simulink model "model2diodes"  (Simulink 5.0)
settings: Solver=ode23t  StartTime=0.0  StopTime=24  FixedStep=0.0001  RelTol=1e-3

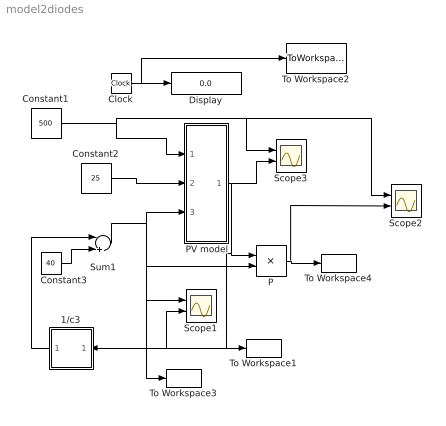
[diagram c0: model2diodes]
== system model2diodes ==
  1/c3 : Subsystem  Orientation=left
  Clock : Clock
  Constant1 : Constant  Value=500
  Constant2 : Constant  Value=25
  Constant3 : Constant  Value=40
  Display : Display
  P : Product
  PV model : Subsystem  mask{p1=0.00345, p2=0.0058e-3, p3=-0.0336e-3, p4=31.2367, Eg=1.76e-19, k=1.38e-23, e0=1.6e-19, a=1, ns=72, rs=0.9225, rsh=235.1551, Eref=1000, Tjref=298}
  Scope1 : Scope  NumInputPorts=2
  Scope2 : Scope  NumInputPorts=2
  Scope3 : Scope  NumInputPorts=2
  Sum1 : Sum  Inputs=|+-
  To Workspace1 : ToWorkspace  VariableName=i  SampleTime=-1  SaveFormat=Array
  To Workspace2 : ToWorkspace  VariableName=t  SampleTime=-1  SaveFormat=Array
  To Workspace3 : ToWorkspace  VariableName=v  SampleTime=-1  SaveFormat=Array
  To Workspace4 : ToWorkspace  VariableName=p  SampleTime=-1  SaveFormat=Array
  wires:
  Constant2/1 -> PV model/2(Ta)
  Constant3/1 -> Sum1/2
  Sum1/1 -> PV model/3(V), P/2, To Workspace3/1, Scope1/1
  P/1 -> Scope2/2, To Workspace4/1
  Clock/1 -> Display/1, To Workspace2/1
  PV model/1(I1) -> Scope3/2, P/1, To Workspace1/1, Scope1/2, 1/c3/1(Idc)
  Constant1/1 -> PV model/1(Es), Scope3/1, Scope2/1
  1/c3/1(Vdc) -> Sum1/1

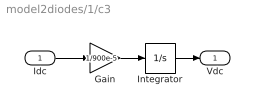
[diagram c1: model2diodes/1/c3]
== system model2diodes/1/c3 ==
  Idc : Inport
  Gain : Gain  Gain=1/900e-5
  Integrator : Integrator
  Vdc : Outport
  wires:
  Gain/1 -> Integrator/1
  Idc/1 -> Gain/1
  Integrator/1 -> Vdc/1

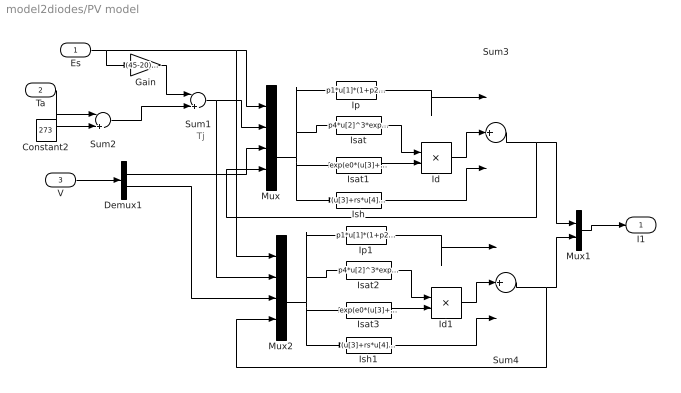
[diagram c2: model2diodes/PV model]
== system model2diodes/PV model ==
  note: Tj
  Es : Inport
  Ta : Inport  Port=2
  V : Inport  Port=3
  Constant2 : Constant  Value=273
  Demux1 : Demux  Outputs=2
  Gain : Gain  Gain=(45-20)/800
  Id : Product
  Id1 : Product
  Ip : Fcn  Expr=p1*u[1]*(1+p2*(u[1]-Eref)+p3*(u[2]-Tjref))
  Ip1 : Fcn  Expr=p1*u[1]*(1+p2*(u[1]-Eref)+p3*(u[2]-Tjref))
  Isat : Fcn  Expr=p4*u[2]^3*exp(-Eg/(k*u[2]))
  Isat1 : Fcn  Expr=exp(e0*(u[3]+rs*u[4])/(a*ns*k*u[2]))-1
  Isat2 : Fcn  Expr=p4*u[2]^3*exp(-Eg/(k*u[2]))
  Isat3 : Fcn  Expr=exp(e0*(u[3]+rs*u[4])/(a*ns*k*u[2]))-1
  Ish : Fcn  Expr=(u[3]+rs*u[4])/rsh
  Ish1 : Fcn  Expr=(u[3]+rs*u[4])/rsh
  Mux : Mux
  Mux1 : Mux  Inputs=2
  Mux2 : Mux
  Sum1 : Sum  Inputs=|++
  Sum2 : Sum  Inputs=|++
  Sum3 : Sum  Inputs=|+--
  Sum4 : Sum  Inputs=|+--
  I1 : Outport
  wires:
  Es/1 -> Gain/1, Mux/1, Mux2/1
  Gain/1 -> Sum1/1
  Constant2/1 -> Sum2/2
  Isat/1 -> Id/1
  Isat1/1 -> Id/2
  Mux/1 -> Ip/1, Isat/1, Isat1/1, Ish/1
  Id/1 -> Sum3/2
  Ip/1 -> Sum3/1
  Ish/1 -> Sum3/3
  Sum3/1 -> Mux/4, Mux1/1
  Ta/1 -> Sum2/1
  V/1 -> Demux1/1
  Demux1/1 -> Mux/3
  Isat2/1 -> Id1/1
  Isat3/1 -> Id1/2
  Mux2/1 -> Ish1/1, Isat3/1, Isat2/1, Ip1/1
  Id1/1 -> Sum4/2
  Ip1/1 -> Sum4/1
  Ish1/1 -> Sum4/3
  Sum4/1 -> Mux2/4, Mux1/2
  Demux1/2 -> Mux2/3
  Mux1/1 -> I1/1
  Sum2/1 -> Sum1/2
  Sum1/1 -> Mux/2, Mux2/2
